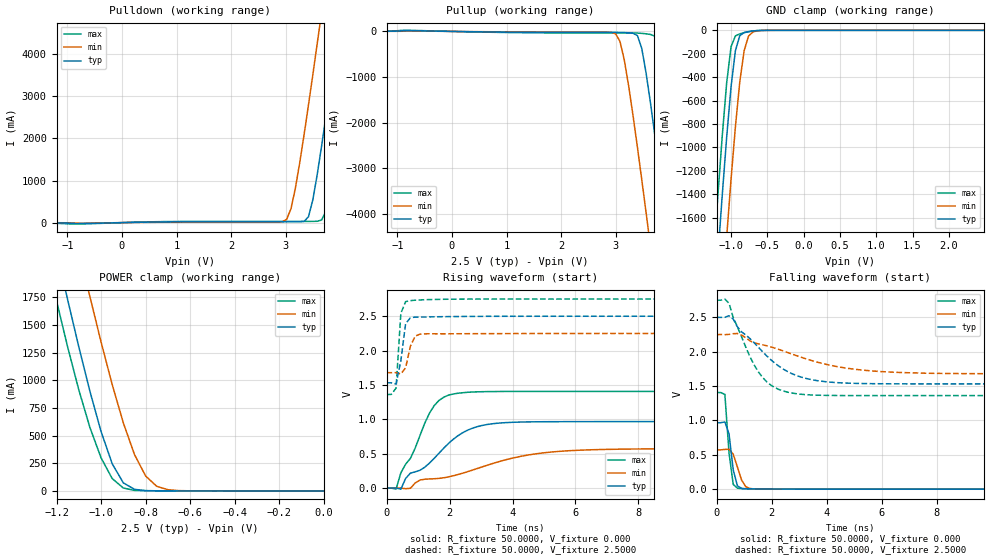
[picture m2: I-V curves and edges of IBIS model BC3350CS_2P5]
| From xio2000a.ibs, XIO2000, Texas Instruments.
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|   Model BC3350CS_2P5
[Model]   BC3350CS_2P5
Model_type   I/O
Enable   Active-Low
Polarity   Non-Inverting
Vinh =   1.75V
Vinl =   0.75V
Vmeas =   1.25V
Cref =   15.0pF
Rref =   100M
Vref =   0.00V
|   typ   min   max
C_comp   1.65pF   1.67pF   1.63pF
[Model Spec]
|   typ   min   max
Vinh   1.750V   1.575V   1.925V
Vinl   0.750V   0.675V   0.825V
Vmeas   1.250V   1.125V   1.375V
[Temperature Range]   25.0   125.0   -40.0
[Voltage Range]   2.50V   2.25V   2.75V
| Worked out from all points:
|   slope of the pulldown table from 0 to 0.375 V, typ, clamps not added: 37.2 ohm
|   slope of the pullup table from 0 to 0.375 V, typ, clamps not added: 52.5 ohm
|   GND clamp passes 1 mA (typ) near -0.59 V on its own axis
|   POWER clamp passes 1 mA (typ) near -0.75 V on its own axis
|   rising waveform, R_fixture 50.0000, V_fixture 0.000: 20-80 % time 1.6ns typ, 3.17ns min, 885ps max; typ from 0 V to 0.967 V
|   rising waveform, R_fixture 50.0000, V_fixture 2.5000: 20-80 % time 184ps typ, 205ps min, 116ps max; typ from 1.53 V to 2.5 V
|   falling waveform, R_fixture 50.0000, V_fixture 0.000: 20-80 % time 200ps typ, 291ps min, 187ps max; typ from 0.967 V to 0 V
|   falling waveform, R_fixture 50.0000, V_fixture 2.5000: 20-80 % time 1.64ns typ, 2.91ns min, 1.01ns max; typ from 2.5 V to 1.53 V
| (Vdd votage range)   1.50V   1.35V   1.65V
| (Process strength)   nominal   weak   strong
[Pulldown]
| voltage   I(typ)   I(min)   I(max)
-2.5V     -466uA     -354uA     -521uA
3.02V     20.28mA    78.74mA    28.88mA
3.18V     20.72mA    820mA      28.96mA
3.42V     139.6mA    2.795A     29.51mA
3.58V     1.141A     4.251A     31.81mA
3.66V     1.816A     4.995A     62.2mA
3.74V     2.528A     5.747A     270.5mA
3.82V     3.261A     6.505A     711.6mA
3.98V     4.761A     8.032A     1.98A
4.22V     7.057A     10.35A     4.181A
4.3V      7.83A      11.12A     4.94A
4.94V     14.08A     17.37A     11.15A
[Pullup]
| voltage   I(typ)   I(min)   I(max)
-2.44V    385uA      291uA      478uA
3V        -22.08mA   -51.51mA   -34.04mA
3.16V     -25.27mA   -625.8mA   -34.21mA
3.4V      -89.75mA   -2.534A    -36.64mA
3.48V     -371.2mA   -3.248A    -42.55mA
3.56V     -915.3mA   -3.978A    -52.64mA
3.72V     -2.272A    -5.468A    -104.1mA
3.8V      -2.999A    -6.223A    -394.8mA
3.96V     -4.493A    -7.748A    -1.665A
4.2V      -6.786A    -10.06A    -3.888A
4.28V     -7.558A    -10.83A    -4.652A
5V        -14.59A    -17.86A    -11.66A
[GND_clamp]
| voltage   I(typ)   I(min)   I(max)
-2.5V     -14.59A    -15.41A    -14.12A
-1.24V    -2.45A     -3.337A    -1.93A
-1.18V    -1.914A    -2.798A    -1.398A
-1.12V    -1.397A    -2.27A     -892.6mA
-1.06V    -910.1mA   -1.759A    -445.6mA
-1V       -481.8mA   -1.271A    -140.2mA
-940mV    -173.6mA   -822.9mA   -47.69mA
-880mV    -46.22mA   -441.6mA   -30.2mA
-820mV    -18.89mA   -174.6mA   -20.09mA
-760mV    -10.58mA   -50.13mA   -11.81mA
-700mV    -5.579mA   -14.05mA   -5.6mA
2.48V     147.9pA    201.8nA    128.2pA
[POWER_clamp]
| voltage   I(typ)   I(min)   I(max)
-2.5V     14.67A     15.51A     14.2A
-1.2V     2.167A     3.062A     1.716A
-1.15V    1.727A     2.616A     1.3A
-1.05V    899.2mA    1.754A     572.6mA
-1V       536.3mA    1.345A     298.8mA
-950mV    245.3mA    960.6mA    111.5mA
-900mV    72.81mA    614.2mA    26.23mA
-850mV    14.59mA    328.9mA    4.932mA
-800mV    2.989mA    135.1mA    1.575mA
-750mV    997.4uA    41.7mA     924.5uA
-650mV    310.2uA    2.816mA    338.3uA
0V        151.2pA    2.389nA    148.3pA
[Ramp]
| variable   typ   min   max
dV/dt_r   0.5802/1.5808n   0.3432/3.1335n   0.8437/0.8760n
dV/dt_f   0.5811/1.6275n   0.3427/2.8835n   0.8330/1.0002n
R_load = 50.0000
[Rising Waveform]
R_fixture = 50.0000
V_fixture = 0.000
V_fixture_min = 0.000
V_fixture_max = 0.000
| time   V(typ)   V(min)   V(max)
0s        1.049nV    28.27nV    530.3pV
303ps     1.175mV    744.3uV    -15.23mV
454.5ps   -15.95mV   515.7uV    221.2mV
757.6ps   216.5mV    -3.503mV   431.7mV
1.061ns   259.1mV    116.4mV    763.2mV
1.515ns   433.3mV    135.6mV    1.201V
2.121ns   710.9mV    179mV      1.369V
3.182ns   923.9mV    330.1mV    1.403V
5.606ns   966.3mV    538mV      1.406V
15ns      967mV      571.9mV    1.406V
[Rising Waveform]
R_fixture = 50.0000
V_fixture = 2.5000
V_fixture_min = 2.2500
V_fixture_max = 2.7500
| time   V(typ)   V(min)   V(max)
0s        1.532V     1.679V     1.362V
151.5ps   1.532V     1.679V     1.362V
303ps     1.514V     1.679V     1.455V
454.5ps   1.852V     1.659V     2.542V
606.1ps   2.393V     1.749V     2.713V
757.6ps   2.478V     2.063V     2.727V
909.1ps   2.488V     2.21V      2.734V
1.061ns   2.488V     2.239V     2.737V
1.212ns   2.489V     2.244V     2.74V
15ns      2.5V       2.25V      2.75V
[Falling Waveform]
R_fixture = 50.0000
V_fixture = 0.000
V_fixture_min = 0.000
V_fixture_max = 0.000
| time   V(typ)   V(min)   V(max)
0s        967mV      571.9mV    1.406V
151.5ps   967mV      571.9mV    1.406V
303ps     978.9mV    578.6mV    1.379V
454.5ps   802mV      580.5mV    523.6mV
606.1ps   279.6mV    508mV      68.47mV
757.6ps   48.31mV    322.4mV    14.91mV
909.1ps   11.67mV    132.8mV    7.459mV
1.061ns   6.293mV    35.84mV    5.189mV
1.364ns   3.93mV     4.242mV    2.811mV
15ns      344.8nV    268.3nV    259.5nV
[Falling Waveform]
R_fixture = 50.0000
V_fixture = 2.5000
V_fixture_min = 2.2500
V_fixture_max = 2.7500
| time   V(typ)   V(min)   V(max)
0s        2.5V       2.25V      2.75V
303ps     2.502V     2.249V     2.766V
454.5ps   2.523V     2.252V     2.703V
606.1ps   2.475V     2.262V     2.498V
1.212ns   2.192V     2.159V     1.929V
1.667ns   2.002V     2.101V     1.628V
2.576ns   1.712V     1.989V     1.412V
3.788ns   1.572V     1.835V     1.366V
5.909ns   1.534V     1.713V     1.362V
15ns      1.532V     1.679V     1.362V
